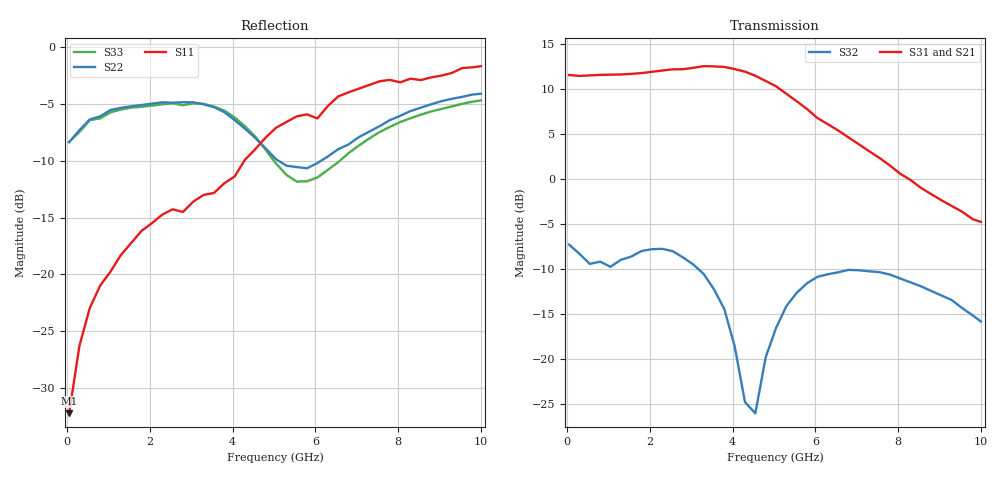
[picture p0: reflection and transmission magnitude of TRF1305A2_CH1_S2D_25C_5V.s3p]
! Created Thu Jun 26 19:35:44 2025
# hz S ma R 50
! 3 Port Network Data from SP1.SP block
! PORT[1] = INP
! PORT[2]= OUTM
! PORT[3] = OUTP
! freq  magS11  angS11  magS12  angS12  magS13  angS13
!  magS21  angS21
!  magS22  angS22  magS23  angS23
!  magS31  angS31  magS32  angS32
!  magS33  angS33
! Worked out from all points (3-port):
!   41 points, 50 MHz to 10 GHz, reference 50 ohm
!   strongest paths, dB at 50 MHz, 2.55 GHz, 5.05 GHz, 7.55 GHz, 10 GHz:
!     S31: 11.5, 12.1, 10.3, 2.3, -4.8
!     S21: 11.5, 12.1, 10.3, 2.5, -4.4
!     S32: -7.3, -8.0, -16.6, -10.4, -15.9
!   lowest |S11| = -32.2 dB at 50 MHz (marker M1), VSWR 1.05, Z = 47.7 - j0.772 ohm
!   |S11| at or under -10 dB: start of sweep to 4.284 GHz
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5e7  0.02445 -160.7  0.00411 33.1  0.002821 -174.6
     3.739 177.7  0.3818 176.3  0.4297 0.5
     3.763 -2.1  0.4305 0.8  0.3828 176.1
1.3e9  0.1216 -120.0  0.02745 27.8  0.01357 11.8
       3.811 131.5  0.5405 125.6  0.3585 -4.4
       3.788 -48.1  0.3544 -5.0  0.5317 127.0
2.55e9  0.1934 -127.8  0.0398 9.3  0.01501 -30.7
        4.03 82.3  0.5694 77.3  0.4074 -32.9
        4.045 -96.9  0.3962 -31.4  0.5667 78.8
3.3e9  0.2238 -123.9  0.05145 -0.6  0.009533 -58.6
       4.206 49.2  0.5607 51.8  0.3106 -56.7
       4.212 -130.4  0.2961 -55.0  0.563 54.2
3.8e9  0.2518 -119.0  0.06201 -11.7  0.007102 -52.6
       4.161 23.9  0.5175 35.7  0.2009 -75.1
       4.171 -155.7  0.1889 -68.9  0.5261 37.5
4.55e9  0.3559 -120.2  0.07777 -37.3  0.01102 -28.0
        3.74 -15.0  0.3984 20.7  0.02554 47.8
        3.727 165.0  0.04984 9.5  0.4037 18.0
5.05e9  0.4418 -129.7  0.08125 -54.3  0.01378 -44.4
        3.256 -39.6  0.3213 20.3  0.1575 44.1
        3.257 139.6  0.1484 30.4  0.3076 14.7
5.8e9  0.506 -150.3  0.07876 -85.0  0.01285 -80.4
       2.455 -72.8  0.2931 30.6  0.2742 19.1
       2.435 106.3  0.2629 16.2  0.2569 30.8
6.8e9  0.6328 -166.4  0.06985 -107.3  0.01336 -101.8
       1.708 -107.2  0.3729 35.9  0.3227 -5.9
       1.695 70.5  0.3117 -6.1  0.3415 40.3
1e10  0.825 148.8  0.04803 -162.2  0.01205 -176.3
      0.6007 168.5  0.6238 -0.8  0.174 -43.5
      0.5756 -19.1  0.1611 -44.9  0.5832 3.3
